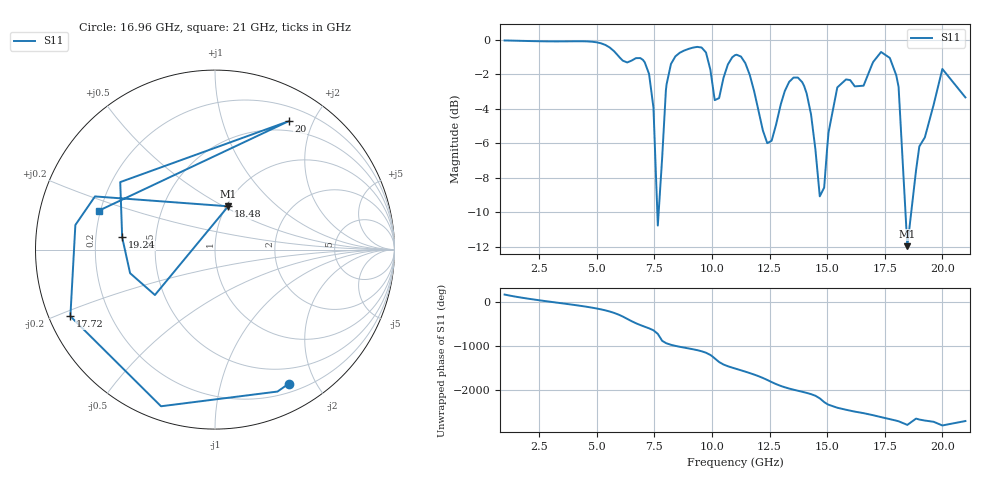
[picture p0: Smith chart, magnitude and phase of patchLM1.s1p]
# GHZ S RI R 50
!Output file by EM3DS_4.0
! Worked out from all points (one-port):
!   107 points, 1 GHz to 21 GHz, reference 50 ohm
!   lowest |S11| = -12.0 dB at 18.48 GHz (marker M1), VSWR 1.67, Z = 51.1 + j26.3 ohm
!   |S11| at or under -10 dB: 7.629 GHz to 7.687 GHz (58.2 MHz wide, 0.76 % of centre); 18.4 GHz to 18.65 GHz (249.7 MHz wide, 1.35 % of centre)
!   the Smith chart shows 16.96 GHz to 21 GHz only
!   S11 on the Smith chart (normalised r, x): 16.96 GHz: 0.30, -1.65; 17.72 GHz: 0.06, -0.22; 18.48 GHz: 1.02, +0.53; 19.24 GHz: 0.32, +0.06; 20 GHz: 0.37, +1.66; 21 GHz: 0.19, +0.16
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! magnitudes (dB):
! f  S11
! 1 GHz  0.0
! 3.66 GHz  -0.1
! 6 GHz  -1.0
! 7.27 GHz  -2.0
! 7.46 GHz  -3.9
! 7.65 GHz  -10.8
! 8.03 GHz  -2.6
! 8.6 GHz  -0.7
! 9.74 GHz  -0.7
! 10.12 GHz  -3.5
! 11 GHz  -0.9
! 11.64 GHz  -2.0
! 12.4 GHz  -6.0
! 13.54 GHz  -2.2
! 14.11 GHz  -3.1
! 14.68 GHz  -9.1
! 14.87 GHz  -8.6
! 15.06 GHz  -5.4
! 15.44 GHz  -2.8
! 16 GHz  -2.3
! 16.96 GHz  -1.4
! 17.72 GHz  -1.0
! 18.1 GHz  -2.7
! 18.48 GHz  -12.0
! 18.86 GHz  -7.5
! 19.24 GHz  -5.7
! 20 GHz  -1.7
! 21 GHz  -3.3
